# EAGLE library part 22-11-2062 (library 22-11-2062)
2.54mm,header,KK,vert,Au,frictn lock,6w Molex KK Series, Series Number 6373, 2.54mm Pitch 6 Way 1 Row Straight PCB Header, Solder Termination Source: Datasheet
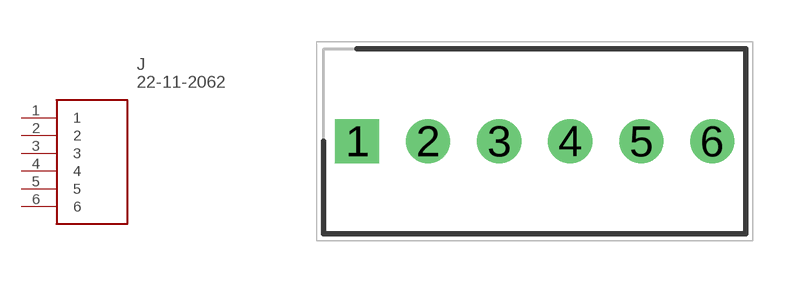
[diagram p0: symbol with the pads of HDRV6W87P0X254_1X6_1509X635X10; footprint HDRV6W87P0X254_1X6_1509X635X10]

Designator prefix J

## 22-11-2062 (Description: 2.54mm,header,KK,vert,Au,frictn lock,6w Molex KK Series, Series Number 6373, 2.54mm Pitch 6 Way 1 Row Straight PCB Header, Solder Termination; Height: 10.92mm; Manufacturer_Name: Molex; Manufacturer_Part_Number: 22-11-2062; Mouser_Part_Number: 538-22-11-2062; Mouser_Price-Stock: https://www.mouser.co.uk/ProductDetail/Molex/22-11-2062?qs=P7cO%252B%252BFDLzRTJGp6b0JM3g%3D%3D)  [HDRV6W87P0X254_1X6_1509X635X10]
1  1
2  2
3  3
4  4
5  5
6  6

## Footprint HDRV6W87P0X254_1X6_1509X635X10 (pad centres in mm)
22-11-2062
drill 1.05 pad 1.575 square: 1 0,0
drill 1.05 pad 1.575: 2 2.54,0; 3 5.08,0; 4 7.62,0; 5 10.16,0; 6 12.7,0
